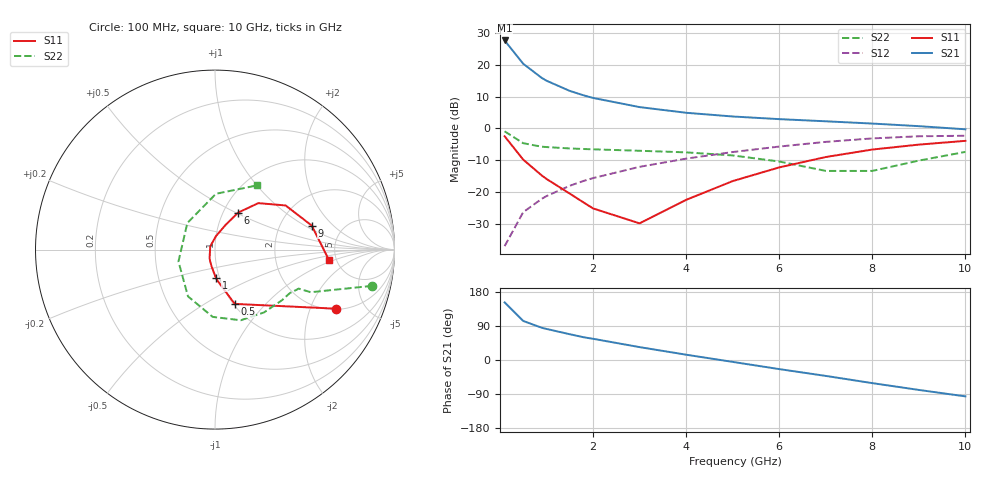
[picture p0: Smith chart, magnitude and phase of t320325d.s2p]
!AT-32032
!S-PARAMETERS at Vce=5V  Ic=10mA.  LAST UPDATED 05-29-98
# ghz s ma r 50
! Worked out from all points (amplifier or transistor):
!   15 points, 100 MHz to 10 GHz, reference 50 ohm
!   highest |S21| = 27.7 dB at 100 MHz (marker M1)
!   |S21| within 3 dB of that: start of sweep to 263.5 MHz
!   unconditionally stable (mu >= 1): 1.013 GHz to 3.057 GHz
!   at 900 MHz: K = 0.99, MSG = 19.0 dB, |S12| = -22.2 dB
!   at 3 GHz: K = 1.00, MAG = 9.1 dB, |S12| = -12.1 dB
!   at 10 GHz: K = 0.91, MSG = 1.0 dB, |S12| = -2.3 dB
!   lowest NFmin = 1.10 dB at 900 MHz
!   S11 on the Smith chart (normalised r, x): 100 MHz: 2.04, -3.08; 500 MHz: 1.01, -0.69; 1 GHz: 0.96, -0.32; 6 GHz: 1.17, +0.51; 9 GHz: 3.00, +1.16; 10 GHz: 4.34, -0.81
0.1  0.751 -26.0  24.17 152.0  0.014 78.0  0.898 -13.0
0.5  0.322 -70.0  10.38 103.0  0.048 68.0  0.584 -24.0
0.9  0.181 -84.0  6.208 85.0  0.078 68.0  0.514 -25.0
1  0.16 -88.0  5.623 82.0  0.086 67.0  0.508 -26.0
1.5  0.094 -102.0  3.885 68.0  0.125 64.0  0.483 -30.0
1.8  0.068 -114.0  3.304 60.0  0.149 61.0  0.473 -34.0
2  0.055 -123.0  3.012 56.0  0.165 59.0  0.468 -37.0
3  0.032 146.0  2.161 34.0  0.248 47.0  0.444 -52.0
4  0.075 86.0  1.759 14.0  0.334 34.0  0.419 -70.0
5  0.148 67.0  1.538 -5.0  0.424 20.0  0.375 -92.0
6  0.243 58.0  1.397 -24.0  0.517 5.0  0.301 -120.0
7  0.354 47.0  1.292 -42.0  0.613 -12.0  0.214 -162.0
8  0.464 32.0  1.19 -61.0  0.695 -31.0  0.214 136.0
9  0.555 14.0  1.083 -79.0  0.751 -51.0  0.311 89.0
10  0.636 -5.0  0.967 -96.0  0.765 -71.0  0.426 57.0
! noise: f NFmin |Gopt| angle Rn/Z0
0.9  1.1  0.29  69  0.2
1.8  1.3  0.25  143  0.12
2  1.4  0.26  159  0.11
2.5  1.5  0.31  -165  0.11
3  1.7  0.37  -133  0.16
3.5  1.9  0.45  -106  0.29
4  2.1  0.52  -84  0.51
